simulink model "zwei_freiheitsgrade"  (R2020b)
settings: Solver=VariableStepAuto  StartTime=0.0  StopTime=10.0  RelTol=1e-6
model workspace (MAT data in the model file):
  c1 = 30
  c2 = 60
  m1 = 3
  m2 = 2

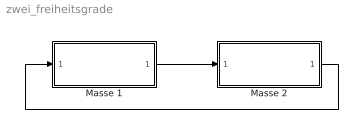
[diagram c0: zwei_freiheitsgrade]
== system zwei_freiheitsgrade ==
  Masse 1 : Subsystem
  Masse 2 : Subsystem
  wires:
  Masse 1/1(x1) -> Masse 2/1(x1)
  Masse 2/1(x2) -> Masse 1/1(x2)

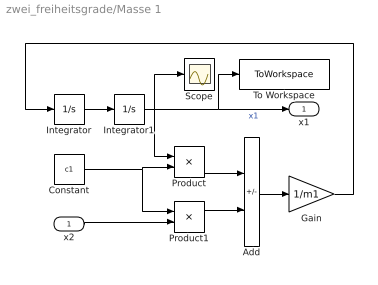
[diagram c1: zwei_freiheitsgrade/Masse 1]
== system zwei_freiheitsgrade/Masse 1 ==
  x2 : Inport
  Add : Sum  Inputs=-+
  Constant : Constant  Value=c1
  Gain : Gain  Gain=1/m1
  Integrator : Integrator
  Integrator1 : Integrator
  Product : Product
  Product1 : Product
  Scope : Scope
  To Workspace : ToWorkspace  VariableName=x1  SaveFormat=Timeseries  SampleTime=-1
  x1 : Outport
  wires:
  Integrator/1 -> Integrator1/1
  Constant/1 -> Product1/1, Product/2
  Integrator1/1 -> To Workspace/1, x1/1, Scope/1, Product/1  "x1"
  Product/1 -> Add/1
  Product1/1 -> Add/2
  x2/1 -> Product1/2
  Add/1 -> Gain/1
  Gain/1 -> Integrator/1

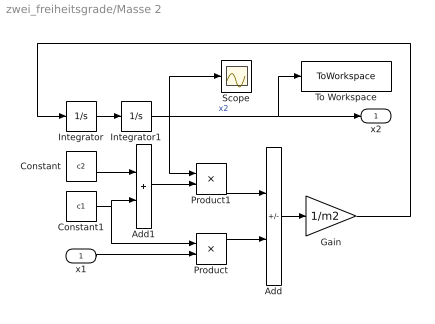
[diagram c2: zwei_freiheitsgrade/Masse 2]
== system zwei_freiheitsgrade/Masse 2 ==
  x1 : Inport
  Add : Sum  Inputs=-+
  Add1 : Sum
  Constant : Constant  Value=c2
  Constant1 : Constant  Value=c1
  Gain : Gain  Gain=1/m2
  Integrator : Integrator
  Integrator1 : Integrator  InitialCondition=0.3
  Product : Product
  Product1 : Product
  Scope : Scope
  To Workspace : ToWorkspace  VariableName=x2  SaveFormat=Timeseries  SampleTime=-1
  x2 : Outport
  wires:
  Integrator/1 -> Integrator1/1
  Constant/1 -> Add1/1
  Constant1/1 -> Product/1, Add1/2
  Add1/1 -> Product1/2
  Add/1 -> Gain/1
  Product/1 -> Add/2
  Product1/1 -> Add/1
  x1/1 -> Product/2
  Integrator1/1 -> To Workspace/1, x2/1, Scope/1, Product1/1  "x2"
  Gain/1 -> Integrator/1
